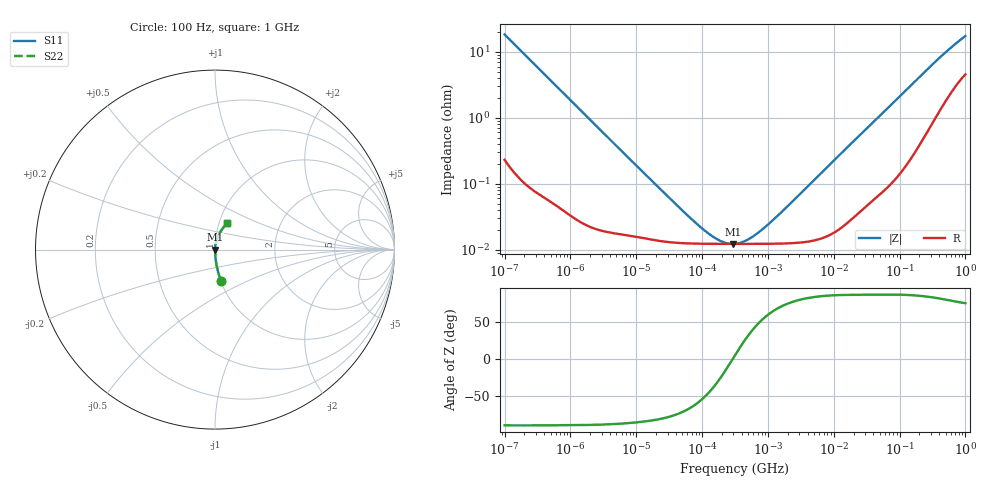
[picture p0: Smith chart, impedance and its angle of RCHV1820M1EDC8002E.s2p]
! RCHV1820M1EDC8002E  S-PARAMETER MODEL  (AEC-Q200 qualified)
! Model Generated by ELNA Corporation (http://www.ty-top.com)
! Version 1.0
! ELNA Control No.240229
! Copyright (c) 2024 ELNA CO.,LTD. All Rights Reserved.
! Products Name : CONDUCTIVE POLYMER HYBRID ALUMINUM ELECTROLYTIC CAPACITORS
! Characteristics :
!  Capacitance  :  82uF  ,  Rated voltage  :  16V
!  Operating Temp. Range  :  -55 to +105 degC  ,  Endurance  :  10000hr at 105 degC
!  Dimension D  :  6.3mm  ,  Dimension L  :  5.8mm
! Frequency Range : 100Hz - 1GHz
! External Node Assignments :
!  1  o---| |---o  2
# MHz S RI R 50
!Freq[MHz].  S11 Real  S11 Imag  S21 Real  S21 Imag  S12 Real  S12 Imag  S22 Real  S22 Imag
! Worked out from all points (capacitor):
!   401 points, 100 Hz to 1 GHz, reference 50 ohm
!   read as one part in series: C = 86.6 uF near 108 Hz
!   lowest |Z| = 12.3 mohm at 291.7 kHz (marker M1)
!   series resonance near 292.5 kHz, so ESL is about 3.4 nH
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0.0001  0.0347 -0.1769  0.9653 0.1769  0.9653 0.1769  0.0347 -0.1769
0.000113  0.0276 -0.158  0.9724 0.158  0.9724 0.158  0.0276 -0.158
0.000183  0.0111 -0.0992  0.9889 0.0992  0.9889 0.0992  0.0111 -0.0992
0.000309  0.00426 -0.0593  0.9957 0.0593  0.9957 0.0593  0.00426 -0.0593
0.001488  0.000413 -0.0125  0.9996 0.0125  0.9996 0.0125  0.000413 -0.0125
0.022131  0.000137 -0.000861  0.9999 0.000861  0.9999 0.000861  0.000137 -0.000861
0.06569  0.000125 -0.000279  0.9999 0.000279  0.9999 0.000279  0.000125 -0.000279
0.120226  0.000123 -0.000134  0.9999 0.000134  0.9999 0.000134  0.000123 -0.000134
0.194984  0.000123 -5.51e-05  0.9999 5.51e-05  0.9999 5.51e-05  0.000123 -5.51e-05
0.238506  0.000123 -2.72e-05  0.9999 2.72e-05  0.9999 2.72e-05  0.000123 -2.72e-05
0.291743  0.000123 -3.42e-07  0.9999 3.42e-07  0.9999 3.42e-07  0.000123 -3.42e-07
0.316228  0.000123 1.03e-05  0.9999 -1.03e-05  0.9999 -1.03e-05  0.000123 1.03e-05
0.386812  0.000123 3.74e-05  0.9999 -3.74e-05  0.9999 -3.74e-05  0.000123 3.74e-05
0.473151  0.000123 6.61e-05  0.9999 -6.61e-05  0.9999 -6.61e-05  0.000123 6.61e-05
0.767361  0.000123 0.000148  0.9999 -0.000148  0.9999 -0.000148  0.000123 0.000148
1.462177  0.000124 0.000317  0.9999 -0.000317  0.9999 -0.000317  0.000124 0.000317
4.704354  0.000138 0.00106  0.9999 -0.00106  0.9999 -0.00106  0.000138 0.00106
69.9842  0.00116 0.0148  0.9988 -0.0148  0.9988 -0.0148  0.00116 0.0148
176.8072  0.00447 0.0365  0.9955 -0.0365  0.9955 -0.0365  0.00447 0.0365
395.8221  0.018 0.0765  0.982 -0.0765  0.982 -0.0765  0.018 0.0765
668.3439  0.0408 0.1152  0.9592 -0.1152  0.9592 -0.1152  0.0408 0.1152
1000  0.0677 0.1497  0.9323 -0.1497  0.9323 -0.1497  0.0677 0.1497
